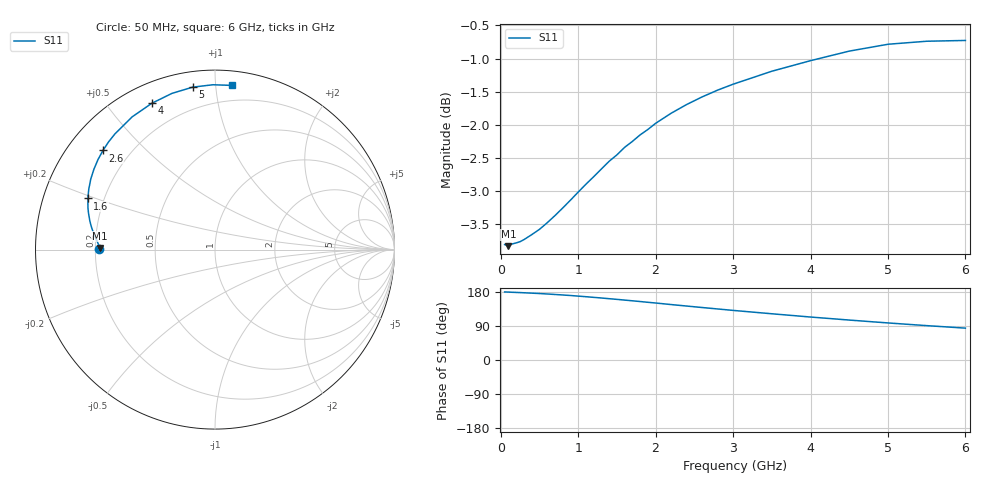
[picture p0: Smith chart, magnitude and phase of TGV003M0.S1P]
! SIEMENS Discrete & RF Semiconductors
! BAT64
! Si Schottky Diode in SOT23
! IF = 3 mA
! S-Parameters:  February  1997
# GHz  S  MA  R  50
!  f  S11
! GHz  MAG  ANG
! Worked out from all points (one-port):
!   34 points, 50 MHz to 6 GHz, reference 50 ohm
!   lowest |S11| = -3.8 dB at 100 MHz (marker M1), VSWR 4.60, Z = 10.9 + j0.333 ohm
!   |S11| at or under -10 dB: nowhere
!   S11 on the Smith chart (normalised r, x): 50 MHz: 0.22, +0.00; 1.6 GHz: 0.14, +0.19; 2.6 GHz: 0.10, +0.38; 4 GHz: 0.08, +0.65; 5 GHz: 0.08, +0.87; 6 GHz: 0.09, +1.10
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0.05  0.6445 179.6
0.1  0.6427 179.2
0.15  0.6452 178.7
0.25  0.6478 177.9
0.3  0.6501 177.4
0.5  0.6618 175.4
0.6  0.6694 174.2
0.8  0.6868 171.6
0.9  0.6963 170.2
1.1  0.7159 167.0
1.2  0.7253 165.3
1.3  0.7352 163.6
1.4  0.7451 161.8
1.5  0.7535 160.0
1.6  0.7635 158.1
1.8  0.7802 154.3
2  0.7961 150.4
2.2  0.8102 146.3
2.4  0.8226 142.4
2.6  0.8336 138.5
2.8  0.8435 134.7
3  0.8522 130.9
3.5  0.8717 122.0
4  0.8879 113.4
4.5  0.9028 105.4
5  0.9136 97.8
5.5  0.9185 90.7
6  0.9197 84.1
